(* Logix 5000 AddOnInstructionDefinition export Banner_R95C8UI_Param_v4; software revision 33.00; part 2 of 2 *)
(* tags used below, declared in another part *)
   R95C : Banner_R95C_8UI_v4;
   Port_Data : Banner_IOL_Port_v4;
   Port : INT;   // Port Number that device is plugged into.
   Local_Control : DINT;
   Command_Being_Processed : BOOL;
   Update_Archive : BOOL;
   Index_Write_Inprocess : DINT;
   Index_Write_Control : DINT;
   Inprocess_Index : DINT;
   Index2 : DINT;
   Index3 : DINT;
(* Banner_R95C8UI_Param_v4, continued *)

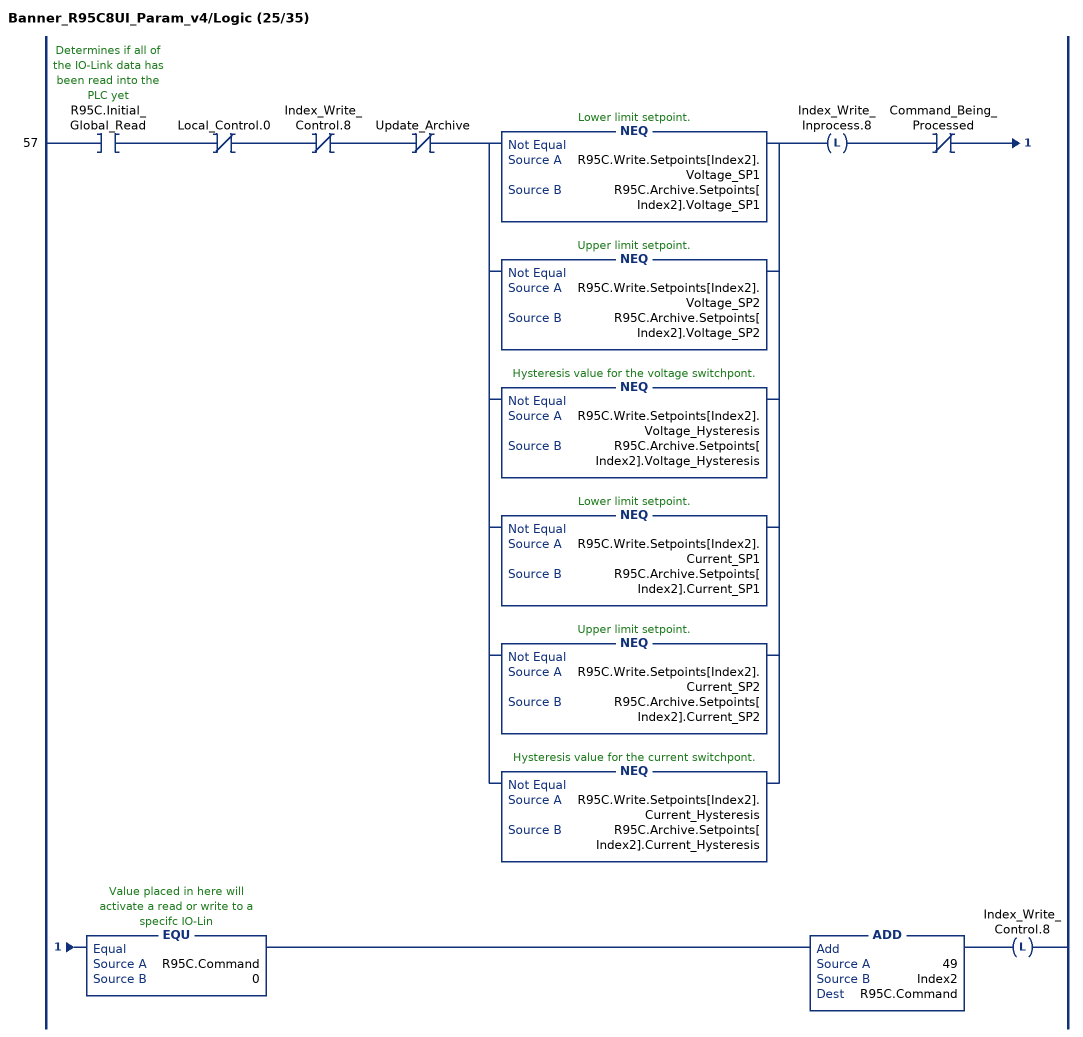
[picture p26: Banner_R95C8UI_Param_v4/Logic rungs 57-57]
   57: XIC(R95C.Initial_Global_Read)XIO(Local_Control.0)XIO(Index_Write_Control.8)XIO(Update_Archive)[NEQ(R95C.Write.Setpoints[Index2].Voltage_SP1,R95C.Archive.Setpoints[Index2].Voltage_SP1) ,NEQ(R95C.Write.Setpoints[Index2].Voltage_SP2,R95C.Archive.Setpoints[Index2].Voltage_SP2) ,NEQ(R95C.Write.Setpoints[Index2].Voltage_Hysteresis,R95C.Archive.Setpoints[Index2].Voltage_Hysteresis) ,NEQ(R95C.Write.Setpoints[Index2].Current_SP1,R95C.Archive.Setpoints[Index2].Current_SP1) ,NEQ(R95C.Write.Setpoints[Index2].Current_SP2,R95C.Archive.Setpoints[Index2].Current_SP2) ,NEQ(R95C.Write.Setpoints[Index2].Current_Hysteresis,R95C.Archive.Setpoints[Index2].Current_Hysteresis) ]OTL(Index_Write_Inprocess.8)XIO(Command_Being_Processed)EQU(R95C.Command,0)ADD(49,Index2,R95C.Command)OTL(Index_Write_Control.8);
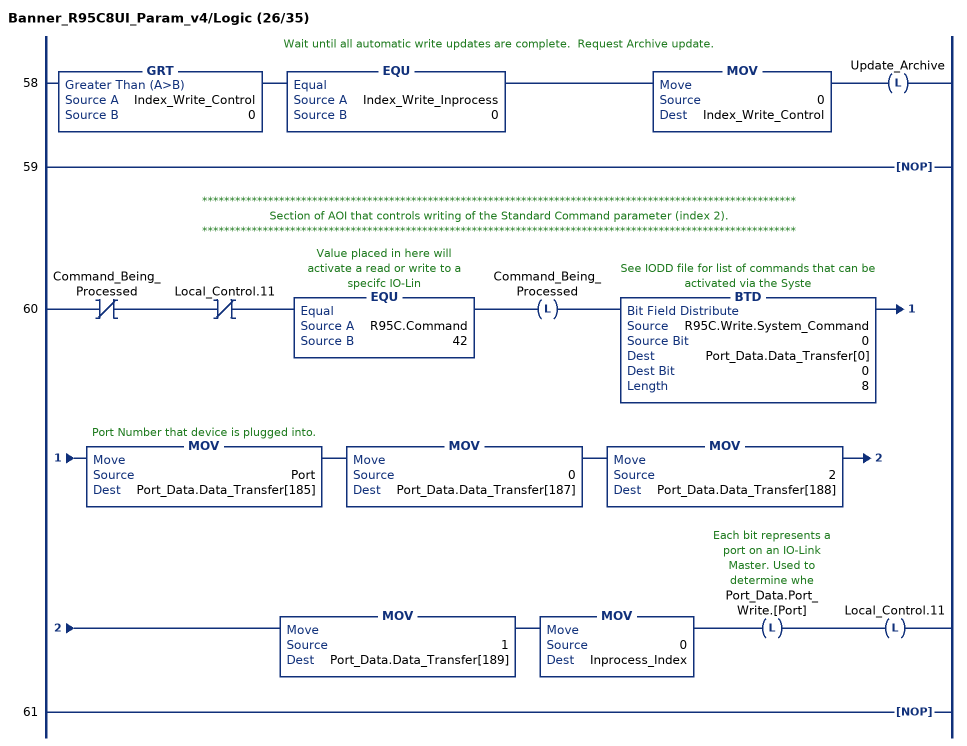
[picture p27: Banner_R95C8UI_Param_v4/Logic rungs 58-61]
   // Wait until all automatic write updates are complete.  Request Archive update.
   58: GRT(Index_Write_Control,0)EQU(Index_Write_Inprocess,0)MOV(0,Index_Write_Control)OTL(Update_Archive);
   59: NOP();
   // ************************************************************************************************************
   // Section of AOI that controls writing of the Standard Command parameter (index 2).
   // ************************************************************************************************************
   60: XIO(Command_Being_Processed)XIO(Local_Control.11)EQU(R95C.Command,42)OTL(Command_Being_Processed)BTD(R95C.Write.System_Command,0,Port_Data.Data_Transfer[0],0,8)MOV(Port,Port_Data.Data_Transfer[185])MOV(0,Port_Data.Data_Transfer[187])MOV(2,Port_Data.Data_Transfer[188])MOV(1,Port_Data.Data_Transfer[189])MOV(0,Inprocess_Index)OTL(Port_Data.Port_Write.[Port])OTL(Local_Control.11);
   61: NOP();
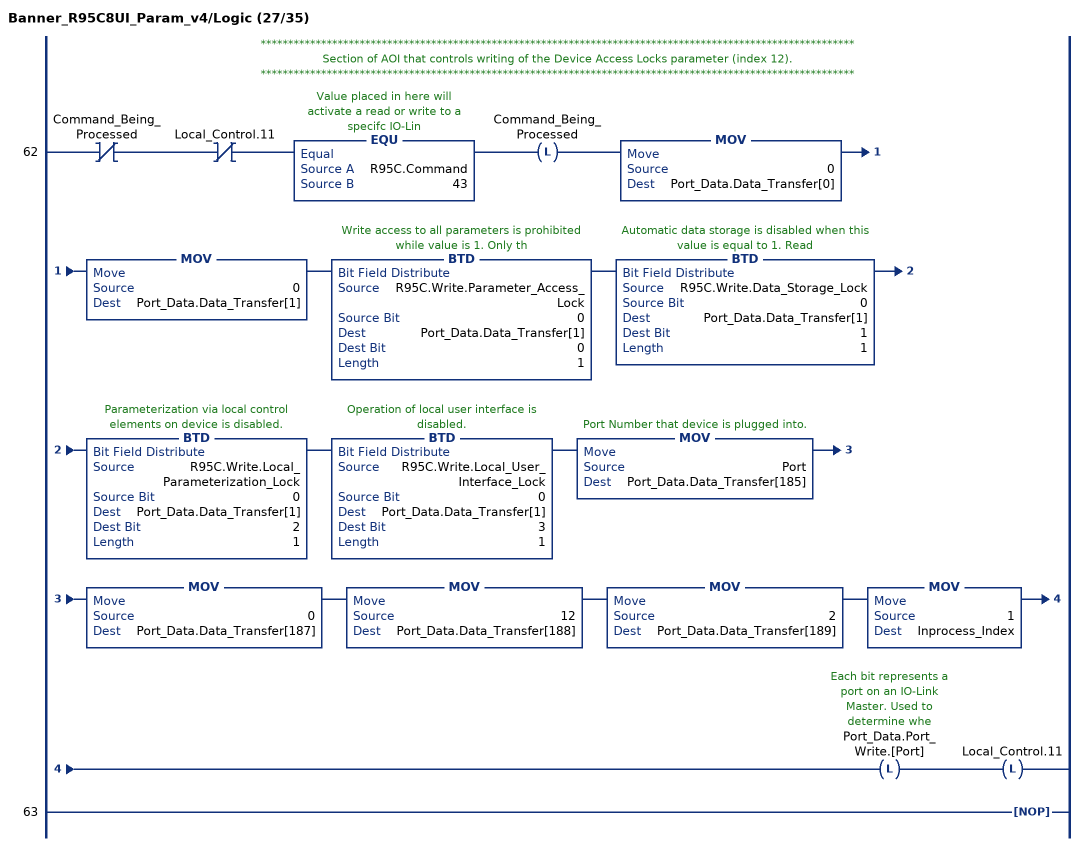
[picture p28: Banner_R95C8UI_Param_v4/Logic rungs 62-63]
   // ************************************************************************************************************
   // Section of AOI that controls writing of the Device Access Locks parameter (index 12).
   // ************************************************************************************************************
   62: XIO(Command_Being_Processed)XIO(Local_Control.11)EQU(R95C.Command,43)OTL(Command_Being_Processed)MOV(0,Port_Data.Data_Transfer[0])MOV(0,Port_Data.Data_Transfer[1])BTD(R95C.Write.Parameter_Access_Lock,0,Port_Data.Data_Transfer[1],0,1)BTD(R95C.Write.Data_Storage_Lock,0,Port_Data.Data_Transfer[1],1,1)BTD(R95C.Write.Local_Parameterization_Lock,0,Port_Data.Data_Transfer[1],2,1)BTD(R95C.Write.Local_User_Interface_Lock,0,Port_Data.Data_Transfer[1],3,1)MOV(Port,Port_Data.Data_Transfer[185])MOV(0,Port_Data.Data_Transfer[187])MOV(12,Port_Data.Data_Transfer[188])MOV(2,Port_Data.Data_Transfer[189])MOV(1,Inprocess_Index)OTL(Port_Data.Port_Write.[Port])OTL(Local_Control.11);
   63: NOP();
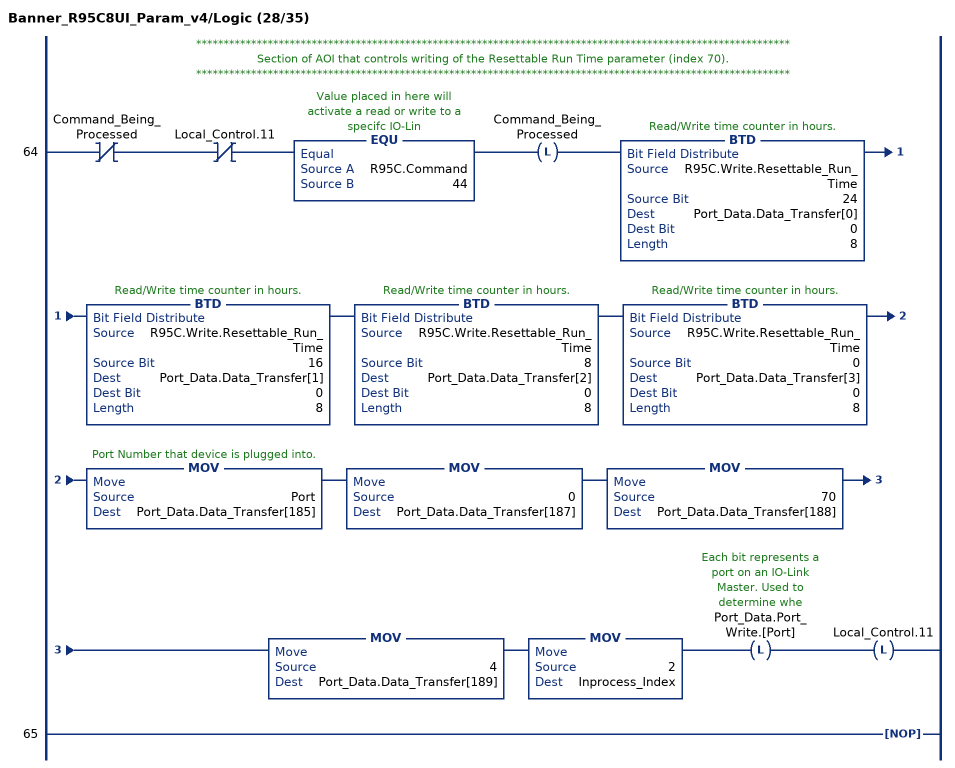
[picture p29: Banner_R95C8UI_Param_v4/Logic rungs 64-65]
   // ************************************************************************************************************
   // Section of AOI that controls writing of the Resettable Run Time parameter (index 70).
   // ************************************************************************************************************
   64: XIO(Command_Being_Processed)XIO(Local_Control.11)EQU(R95C.Command,44)OTL(Command_Being_Processed)BTD(R95C.Write.Resettable_Run_Time,24,Port_Data.Data_Transfer[0],0,8)BTD(R95C.Write.Resettable_Run_Time,16,Port_Data.Data_Transfer[1],0,8)BTD(R95C.Write.Resettable_Run_Time,8,Port_Data.Data_Transfer[2],0,8)BTD(R95C.Write.Resettable_Run_Time,0,Port_Data.Data_Transfer[3],0,8)MOV(Port,Port_Data.Data_Transfer[185])MOV(0,Port_Data.Data_Transfer[187])MOV(70,Port_Data.Data_Transfer[188])MOV(4,Port_Data.Data_Transfer[189])MOV(2,Inprocess_Index)OTL(Port_Data.Port_Write.[Port])OTL(Local_Control.11);
   65: NOP();
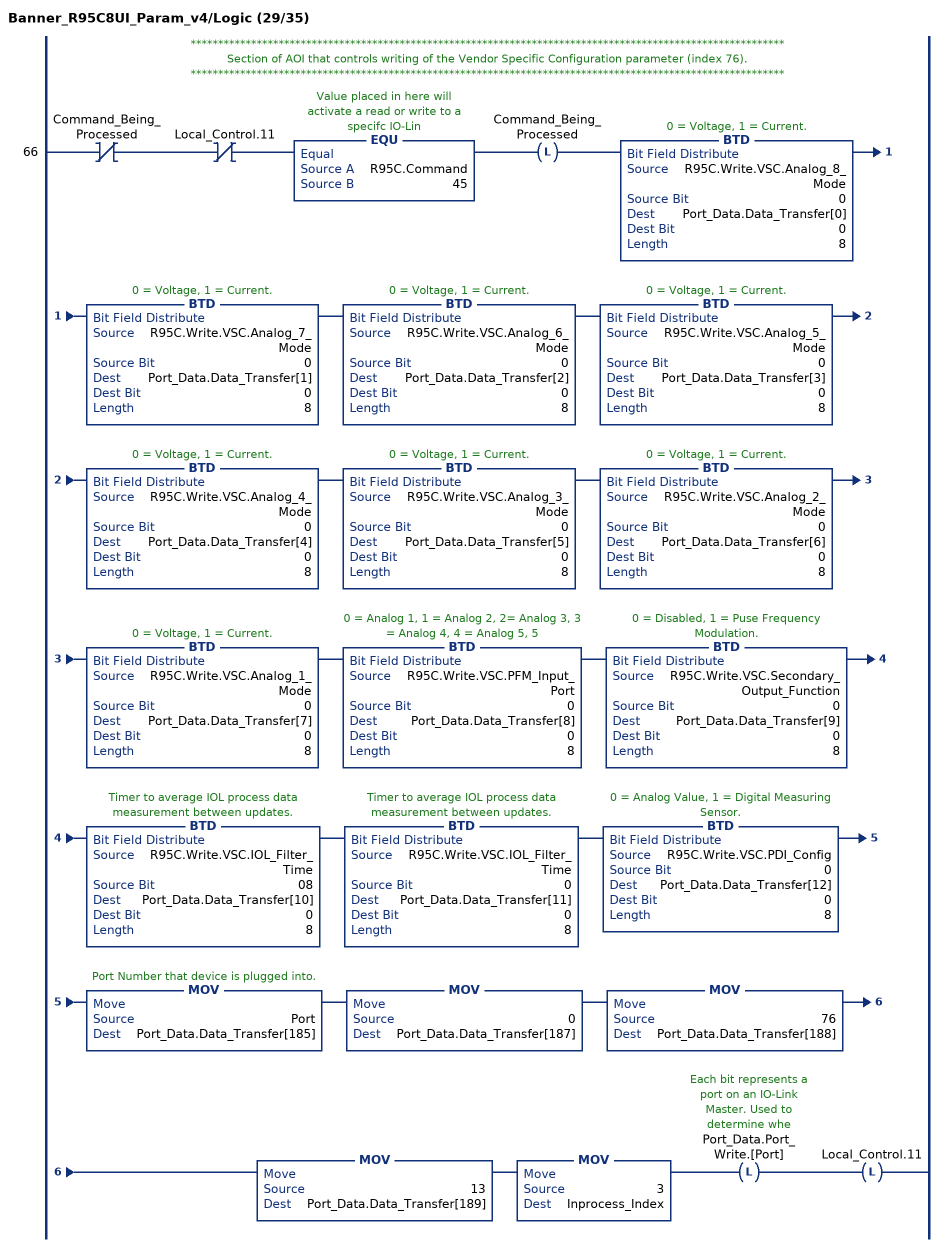
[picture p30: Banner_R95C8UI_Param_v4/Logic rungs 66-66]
   // ************************************************************************************************************
   // Section of AOI that controls writing of the Vendor Specific Configuration parameter (index 76).
   // ************************************************************************************************************
   66: XIO(Command_Being_Processed)XIO(Local_Control.11)EQU(R95C.Command,45)OTL(Command_Being_Processed)BTD(R95C.Write.VSC.Analog_8_Mode,0,Port_Data.Data_Transfer[0],0,8)BTD(R95C.Write.VSC.Analog_7_Mode,0,Port_Data.Data_Transfer[1],0,8)BTD(R95C.Write.VSC.Analog_6_Mode,0,Port_Data.Data_Transfer[2],0,8)BTD(R95C.Write.VSC.Analog_5_Mode,0,Port_Data.Data_Transfer[3],0,8)BTD(R95C.Write.VSC.Analog_4_Mode,0,Port_Data.Data_Transfer[4],0,8)BTD(R95C.Write.VSC.Analog_3_Mode,0,Port_Data.Data_Transfer[5],0,8)BTD(R95C.Write.VSC.Analog_2_Mode,0,Port_Data.Data_Transfer[6],0,8)BTD(R95C.Write.VSC.Analog_1_Mode,0,Port_Data.Data_Transfer[7],0,8)BTD(R95C.Write.VSC.PFM_Input_Port,0,Port_Data.Data_Transfer[8],0,8)BTD(R95C.Write.VSC.Secondary_Output_Function,0,Port_Data.Data_Transfer[9],0,8)BTD(R95C.Write.VSC.IOL_Filter_Time,08,Port_Data.Data_Transfer[10],0,8)BTD(R95C.Write.VSC.IOL_Filter_Time,0,Port_Data.Data_Transfer[11],0,8)BTD(R95C.Write.VSC.PDI_Config,0,Port_Data.Data_Transfer[12],0,8)MOV(Port,Port_Data.Data_Transfer[185])MOV(0,Port_Data.Data_Transfer[187])MOV(76,Port_Data.Data_Transfer[188])MOV(13,Port_Data.Data_Transfer[189])MOV(3,Inprocess_Index)OTL(Port_Data.Port_Write.[Port])OTL(Local_Control.11);
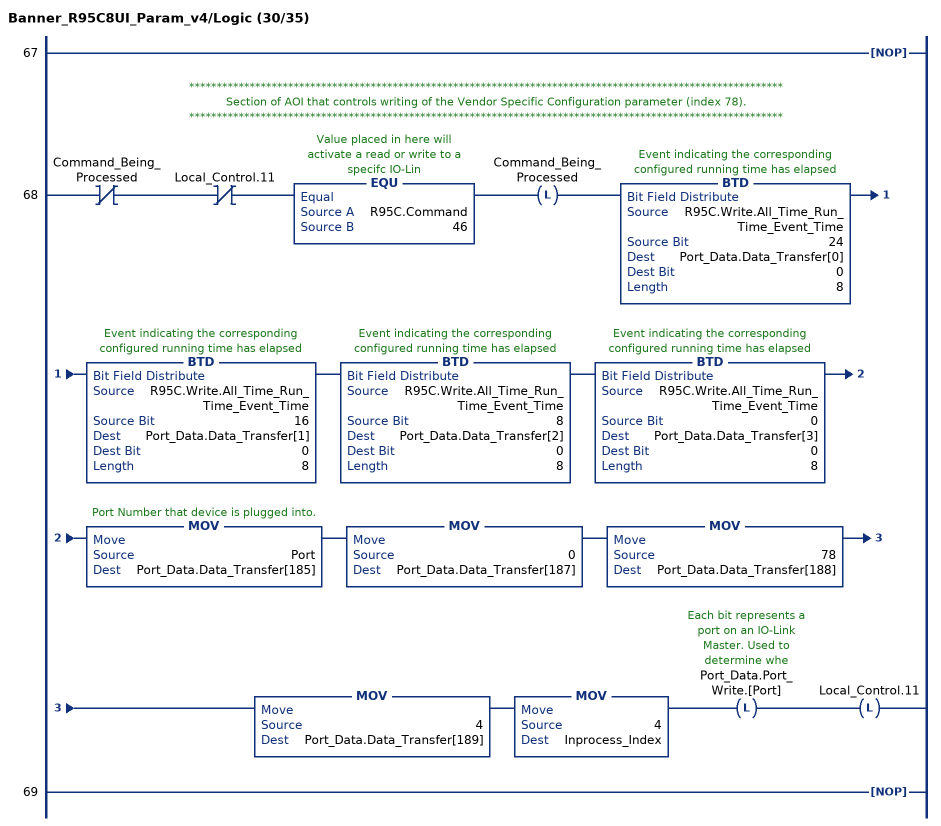
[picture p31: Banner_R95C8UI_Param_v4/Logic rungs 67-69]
   67: NOP();
   // ************************************************************************************************************
   // Section of AOI that controls writing of the Vendor Specific Configuration parameter (index 78).
   // ************************************************************************************************************
   68: XIO(Command_Being_Processed)XIO(Local_Control.11)EQU(R95C.Command,46)OTL(Command_Being_Processed)BTD(R95C.Write.All_Time_Run_Time_Event_Time,24,Port_Data.Data_Transfer[0],0,8)BTD(R95C.Write.All_Time_Run_Time_Event_Time,16,Port_Data.Data_Transfer[1],0,8)BTD(R95C.Write.All_Time_Run_Time_Event_Time,8,Port_Data.Data_Transfer[2],0,8)BTD(R95C.Write.All_Time_Run_Time_Event_Time,0,Port_Data.Data_Transfer[3],0,8)MOV(Port,Port_Data.Data_Transfer[185])MOV(0,Port_Data.Data_Transfer[187])MOV(78,Port_Data.Data_Transfer[188])MOV(4,Port_Data.Data_Transfer[189])MOV(4,Inprocess_Index)OTL(Port_Data.Port_Write.[Port])OTL(Local_Control.11);
   69: NOP();
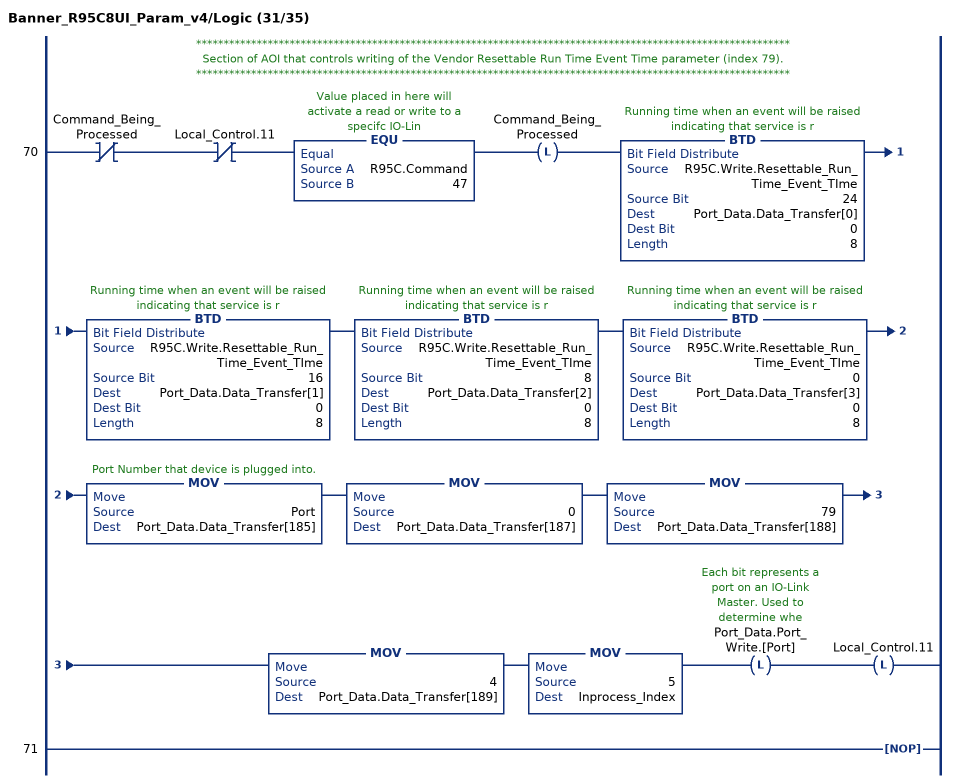
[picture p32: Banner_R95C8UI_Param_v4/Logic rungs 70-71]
   // ************************************************************************************************************
   // Section of AOI that controls writing of the Vendor Resettable Run Time Event Time parameter (index 79).
   // ************************************************************************************************************
   70: XIO(Command_Being_Processed)XIO(Local_Control.11)EQU(R95C.Command,47)OTL(Command_Being_Processed)BTD(R95C.Write.Resettable_Run_Time_Event_TIme,24,Port_Data.Data_Transfer[0],0,8)BTD(R95C.Write.Resettable_Run_Time_Event_TIme,16,Port_Data.Data_Transfer[1],0,8)BTD(R95C.Write.Resettable_Run_Time_Event_TIme,8,Port_Data.Data_Transfer[2],0,8)BTD(R95C.Write.Resettable_Run_Time_Event_TIme,0,Port_Data.Data_Transfer[3],0,8)MOV(Port,Port_Data.Data_Transfer[185])MOV(0,Port_Data.Data_Transfer[187])MOV(79,Port_Data.Data_Transfer[188])MOV(4,Port_Data.Data_Transfer[189])MOV(5,Inprocess_Index)OTL(Port_Data.Port_Write.[Port])OTL(Local_Control.11);
   71: NOP();
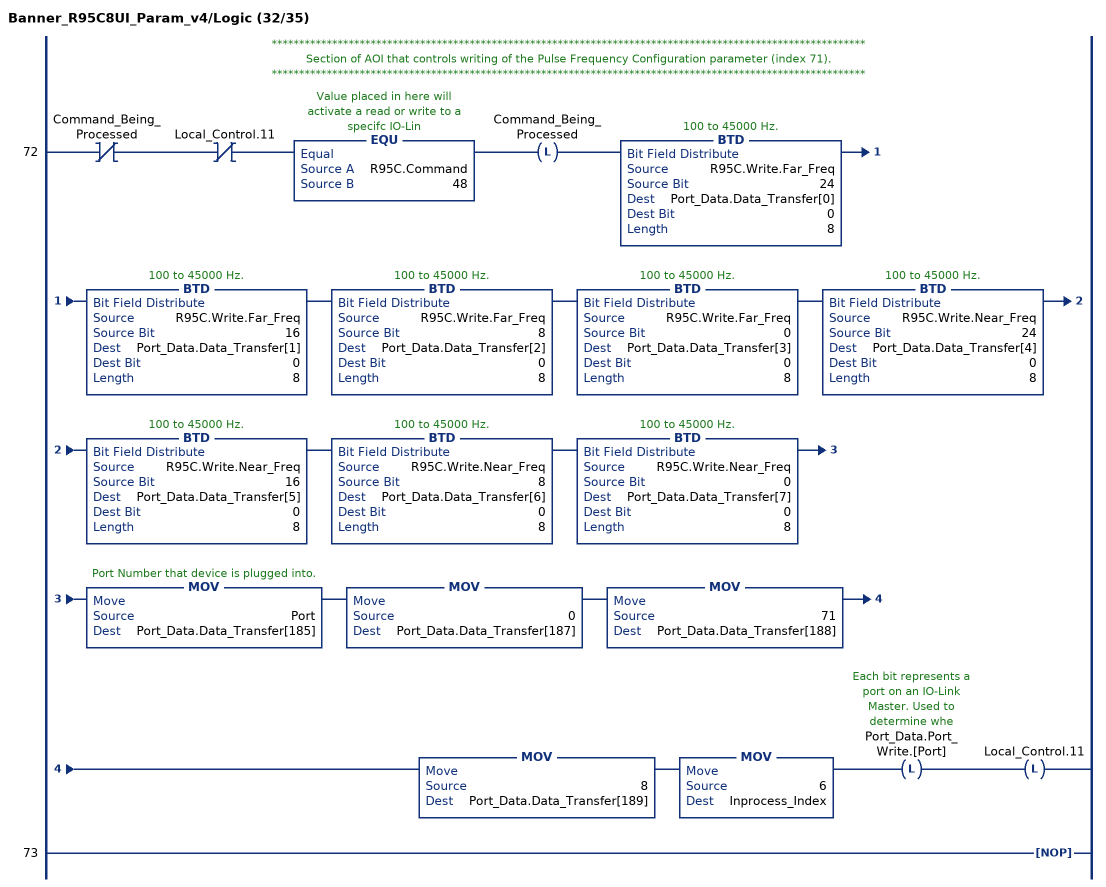
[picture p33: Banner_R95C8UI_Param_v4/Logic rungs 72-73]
   // ************************************************************************************************************
   // Section of AOI that controls writing of the Pulse Frequency Configuration parameter (index 71).
   // ************************************************************************************************************
   72: XIO(Command_Being_Processed)XIO(Local_Control.11)EQU(R95C.Command,48)OTL(Command_Being_Processed)BTD(R95C.Write.Far_Freq,24,Port_Data.Data_Transfer[0],0,8)BTD(R95C.Write.Far_Freq,16,Port_Data.Data_Transfer[1],0,8)BTD(R95C.Write.Far_Freq,8,Port_Data.Data_Transfer[2],0,8)BTD(R95C.Write.Far_Freq,0,Port_Data.Data_Transfer[3],0,8)BTD(R95C.Write.Near_Freq,24,Port_Data.Data_Transfer[4],0,8)BTD(R95C.Write.Near_Freq,16,Port_Data.Data_Transfer[5],0,8)BTD(R95C.Write.Near_Freq,8,Port_Data.Data_Transfer[6],0,8)BTD(R95C.Write.Near_Freq,0,Port_Data.Data_Transfer[7],0,8)MOV(Port,Port_Data.Data_Transfer[185])MOV(0,Port_Data.Data_Transfer[187])MOV(71,Port_Data.Data_Transfer[188])MOV(8,Port_Data.Data_Transfer[189])MOV(6,Inprocess_Index)OTL(Port_Data.Port_Write.[Port])OTL(Local_Control.11);
   73: NOP();
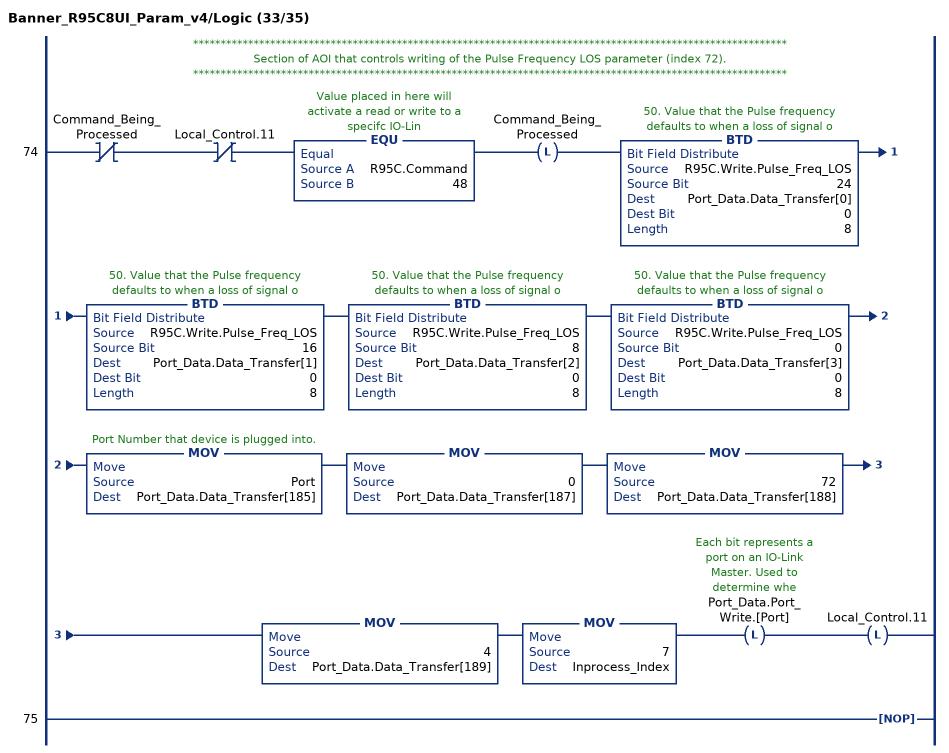
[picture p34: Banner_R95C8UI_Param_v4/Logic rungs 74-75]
   // ************************************************************************************************************
   // Section of AOI that controls writing of the Pulse Frequency LOS parameter (index 72).
   // ************************************************************************************************************
   74: XIO(Command_Being_Processed)XIO(Local_Control.11)EQU(R95C.Command,48)OTL(Command_Being_Processed)BTD(R95C.Write.Pulse_Freq_LOS,24,Port_Data.Data_Transfer[0],0,8)BTD(R95C.Write.Pulse_Freq_LOS,16,Port_Data.Data_Transfer[1],0,8)BTD(R95C.Write.Pulse_Freq_LOS,8,Port_Data.Data_Transfer[2],0,8)BTD(R95C.Write.Pulse_Freq_LOS,0,Port_Data.Data_Transfer[3],0,8)MOV(Port,Port_Data.Data_Transfer[185])MOV(0,Port_Data.Data_Transfer[187])MOV(72,Port_Data.Data_Transfer[188])MOV(4,Port_Data.Data_Transfer[189])MOV(7,Inprocess_Index)OTL(Port_Data.Port_Write.[Port])OTL(Local_Control.11);
   75: NOP();
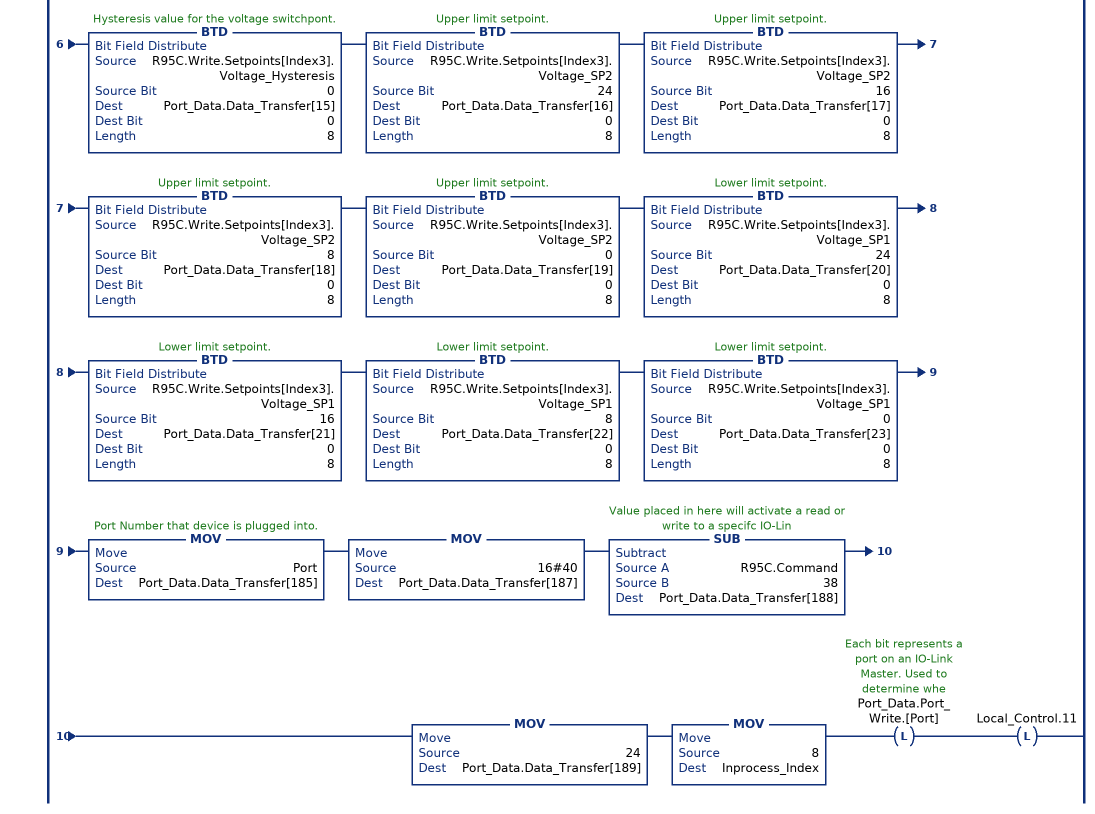
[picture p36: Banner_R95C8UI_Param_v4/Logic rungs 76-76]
   // ************************************************************************************************************
   // Section of AOI that controls writing of the Channel # Setpoints Parameters (index 16396 to Index 16403).
   // ************************************************************************************************************
   76: XIO(Command_Being_Processed)XIO(Local_Control.11)GEQ(R95C.Command,50)LEQ(R95C.Command,57)SUB(R95C.Command,49,Index3)OTL(Command_Being_Processed)BTD(R95C.Write.Setpoints[Index3].Current_Hysteresis,24,Port_Data.Data_Transfer[0],0,8)BTD(R95C.Write.Setpoints[Index3].Current_Hysteresis,16,Port_Data.Data_Transfer[1],0,8)BTD(R95C.Write.Setpoints[Index3].Current_Hysteresis,8,Port_Data.Data_Transfer[2],0,8)BTD(R95C.Write.Setpoints[Index3].Current_Hysteresis,0,Port_Data.Data_Transfer[3],0,8)BTD(R95C.Write.Setpoints[Index3].Current_SP2,24,Port_Data.Data_Transfer[4],0,8)BTD(R95C.Write.Setpoints[Index3].Current_SP2,16,Port_Data.Data_Transfer[5],0,8)BTD(R95C.Write.Setpoints[Index3].Current_SP2,8,Port_Data.Data_Transfer[6],0,8)BTD(R95C.Write.Setpoints[Index3].Current_SP2,0,Port_Data.Data_Transfer[7],0,8)BTD(R95C.Write.Setpoints[Index3].Current_SP1,24,Port_Data.Data_Transfer[8],0,8)BTD(R95C.Write.Setpoints[Index3].Current_SP1,16,Port_Data.Data_Transfer[9],0,8)BTD(R95C.Write.Setpoints[Index3].Current_SP1,8,Port_Data.Data_Transfer[10],0,8)BTD(R95C.Write.Setpoints[Index3].Current_SP1,0,Port_Data.Data_Transfer[11],0,8)BTD(R95C.Write.Setpoints[Index3].Voltage_Hysteresis,24,Port_Data.Data_Transfer[12],0,8)BTD(R95C.Write.Setpoints[Index3].Voltage_Hysteresis,16,Port_Data.Data_Transfer[13],0,8)BTD(R95C.Write.Setpoints[Index3].Voltage_Hysteresis,8,Port_Data.Data_Transfer[14],0,8)BTD(R95C.Write.Setpoints[Index3].Voltage_Hysteresis,0,Port_Data.Data_Transfer[15],0,8)BTD(R95C.Write.Setpoints[Index3].Voltage_SP2,24,Port_Data.Data_Transfer[16],0,8)BTD(R95C.Write.Setpoints[Index3].Voltage_SP2,16,Port_Data.Data_Transfer[17],0,8)BTD(R95C.Write.Setpoints[Index3].Voltage_SP2,8,Port_Data.Data_Transfer[18],0,8)BTD(R95C.Write.Setpoints[Index3].Voltage_SP2,0,Port_Data.Data_Transfer[19],0,8)BTD(R95C.Write.Setpoints[Index3].Voltage_SP1,24,Port_Data.Data_Transfer[20],0,8)BTD(R95C.Write.Setpoints[Index3].Voltage_SP1,16,Port_Data.Data_Transfer[21],0,8)BTD(R95C.Write.Setpoints[Index3].Voltage_SP1,8,Port_Data.Data_Transfer[22],0,8)BTD(R95C.Write.Setpoints[Index3].Voltage_SP1,0,Port_Data.Data_Transfer[23],0,8)MOV(Port,Port_Data.Data_Transfer[185])MOV(16#40,Port_Data.Data_Transfer[187])SUB(R95C.Command,38,Port_Data.Data_Transfer[188])MOV(24,Port_Data.Data_Transfer[189])MOV(8,Inprocess_Index)OTL(Port_Data.Port_Write.[Port])OTL(Local_Control.11);
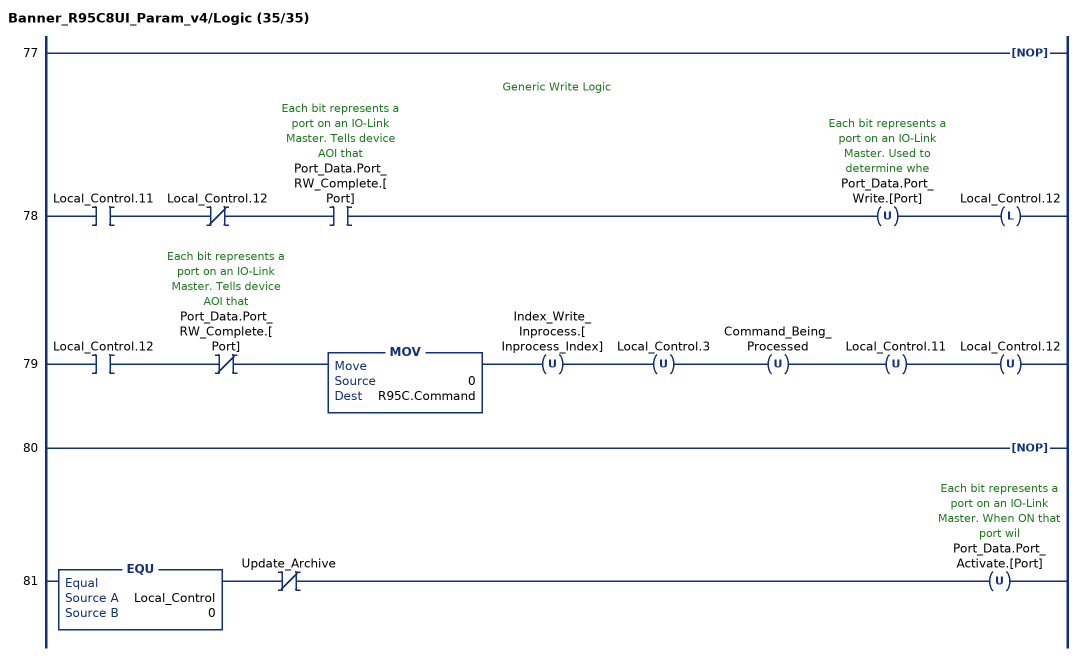
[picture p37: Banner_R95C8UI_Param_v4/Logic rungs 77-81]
   77: NOP();
   // Generic Write Logic
   78: XIC(Local_Control.11)XIO(Local_Control.12)XIC(Port_Data.Port_RW_Complete.[Port])OTU(Port_Data.Port_Write.[Port])OTL(Local_Control.12);
   79: XIC(Local_Control.12)XIO(Port_Data.Port_RW_Complete.[Port])MOV(0,R95C.Command)OTU(Index_Write_Inprocess.[Inprocess_Index])OTU(Local_Control.3)OTU(Command_Being_Processed)OTU(Local_Control.11)OTU(Local_Control.12);
   80: NOP();
   81: EQU(Local_Control,0)XIO(Update_Archive)OTU(Port_Data.Port_Activate.[Port]);
END_ROUTINE
END_ADD_ON_INSTRUCTION
